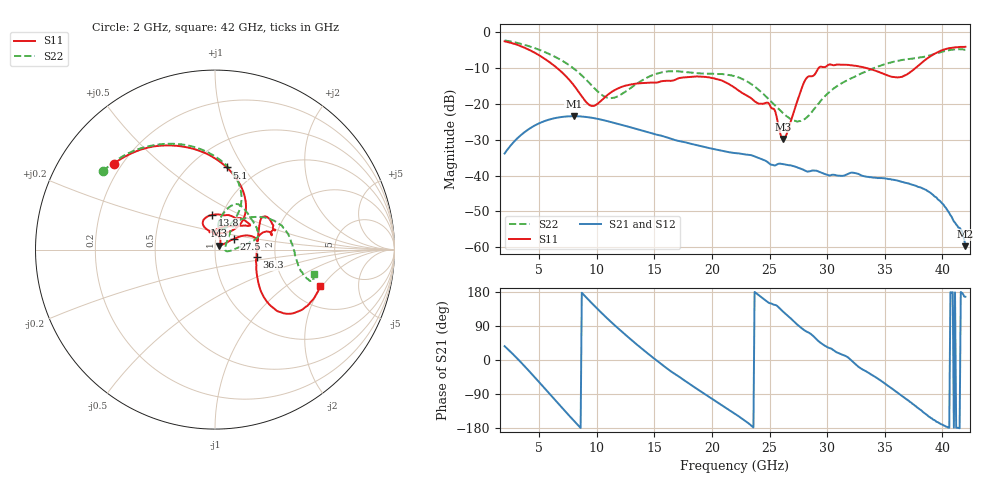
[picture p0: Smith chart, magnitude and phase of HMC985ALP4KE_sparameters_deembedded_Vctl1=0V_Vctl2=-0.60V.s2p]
!s2p File: Measurements: S11, S21, S12, S22
# GHz S dB R 50.0
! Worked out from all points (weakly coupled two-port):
!   401 points, 2 GHz to 42 GHz, reference 50 ohm
!   highest |S21| = -23.47 dB at 8 GHz (marker M1); lowest = -59.7 dB at 42 GHz (marker M2)
!   lowest |S11| = -29.8 dB at 26.2 GHz (marker M3), VSWR 1.07, Z = 52.4 + j2.24 ohm
!   |S11| at or under -10 dB: 6.537 GHz to 29.27 GHz (22.74 GHz wide, 127 % of centre); 33.34 GHz to 37.69 GHz (4.35 GHz wide, 12.2 % of centre)
!   |S22| runs from -25.0 to -2.4 dB; largest |S21 - S12| = 0.00016
!   S11 on the Smith chart (normalised r, x): 2 GHz: 0.17, +0.36; 5.1 GHz: 0.73, +0.85; 13.8 GHz: 0.90, +0.36; 27.5 GHz: 1.22, +0.15; 36.3 GHz: 1.59, -0.14; 42 GHz: 2.90, -1.91
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2  -2.62 139.8  -33.86 36.5  -33.86 36.4  -2.37 145.1
3.5  -4.09 111.9  -28.51 -8.8  -28.51 -8.8  -3.39 121.0
5.1  -6.70 81.9  -25.30 -61.9  -25.31 -62.0  -5.09 96.6
8  -14.82 45.2  -23.47 -159.9  -23.48 -159.9  -10.18 61.6
8.7  -17.95 51.6  -23.56 177.4  -23.57 177.4  -12.11 57.8
9.7  -20.61 86.5  -23.97 145.9  -23.98 145.9  -15.36 58.4
11.1  -17.14 115.3  -24.99 104.3  -24.99 104.3  -18.43 73.8
13.8  -14.27 95.2  -27.35 32.8  -27.34 32.8  -13.75 77.2
15.4  -13.94 73.0  -28.76 -5.6  -28.76 -5.6  -11.43 68.3
19.4  -12.52 34.7  -32.08 -90.4  -32.08 -90.5  -11.60 35.2
22  -15.59 52.2  -33.73 -141.9  -33.75 -141.9  -12.36 15.3
25  -20.21 97.7  -36.76 149.9  -36.77 149.9  -18.99 1.9
26.2  -29.81 41.2  -36.83 126.9  -36.84 126.9  -22.71 -7.4
27.5  -18.41 29.6  -37.86 91.3  -37.84 91.2  -24.89 2.3
28.1  -13.37 20.7  -38.66 76.9  -38.63 76.8  -24.16 18.3
28.7  -12.32 12.8  -38.60 65.8  -38.67 65.8  -22.16 32.5
31  -9.09 23.3  -40.05 18.1  -40.06 17.9  -14.77 52.4
33.3  -9.96 34.4  -40.25 -28.7  -40.26 -28.8  -11.11 40.6
35.4  -12.27 12.4  -41.01 -70.5  -41.01 -70.7  -8.62 25.0
36.3  -12.57 -10.2  -41.59 -90.5  -41.59 -90.6  -7.95 17.5
39.8  -5.31 -41.3  -47.10 -168.0  -47.17 -168.3  -5.65 -16.4
42  -4.14 -19.0  -59.68 166.9  -59.65 163.8  -4.94 -14.1
